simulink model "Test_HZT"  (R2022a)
settings: Solver=VariableStepAuto  StartTime=0.0  StopTime=10.0  RelTol=1e-3

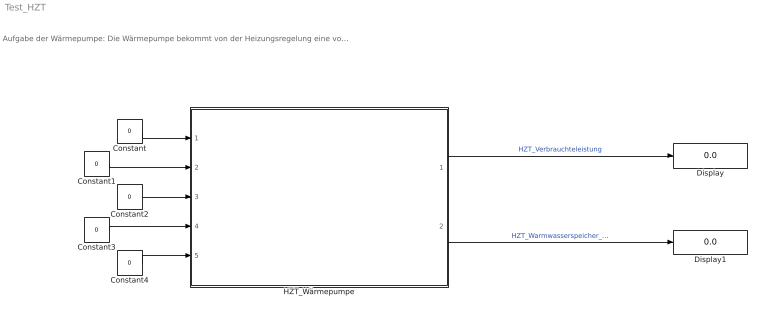
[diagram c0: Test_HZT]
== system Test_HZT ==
  note: Aufgabe der Wärmepumpe: Die Wärmepumpe bekommt von der Heizungsregelung eine vorgegebene Heizleistung, welche in das Haus eingespeist werden soll. Die Leistung wird dann von den Energieerzeugern genommen und umgewandelt. Das gleiche gilt für die Warmwasserheizleistung.
  Constant{,1..4} (5 alike) : Constant  Value=0
  Display : Display
  Display1 : Display
  HZT_Wärmepumpe : Subsystem
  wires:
  HZT_Wärmepumpe/1(HZT_verbrauchte_Leistung) -> Display/1  "HZT_Verbrauchteleistung"
  Constant1/1 -> HZT_Wärmepumpe/2(PAR_LKT_Temperatur)
  Constant4/1 -> HZT_Wärmepumpe/5(ESP_Stromnetz)
  HZT_Wärmepumpe/2(HZT_Warmwasserspeicher_verbrauchte_Leistung) -> Display1/1  "HZT_Warmwasserspeicher_verbrauchte_Leistung"
  Constant/1 -> HZT_Wärmepumpe/1(HZR_Heizleistung)
  Constant2/1 -> HZT_Wärmepumpe/3(HZR_Warmwasserleistung)
  Constant3/1 -> HZT_Wärmepumpe/4(ESP_Strom)

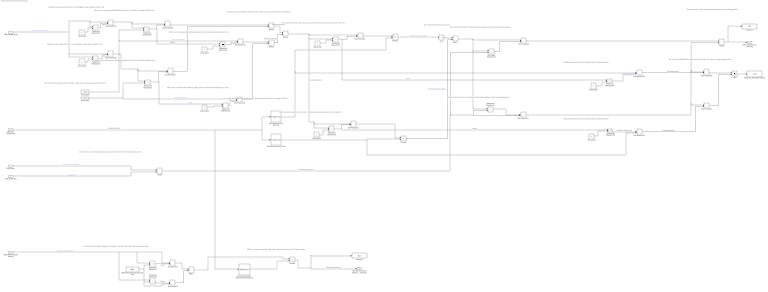
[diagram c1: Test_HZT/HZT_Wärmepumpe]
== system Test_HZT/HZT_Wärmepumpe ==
  note: Summiert alle Leistungen zusammen. (Es kommt nur aus einem Pfad ein tatsächlicher Wert, die anderen ergeben null)
  note: Modul zur berechnung der tatsächlich verbrauchten Energie für Warmwasser
  note: Leistung muss größer nulll sein, um anzugeben, dass geheizt werden soll
  note: Wenn gekühlt werden soll, wird die zu verbrauchende Leistung errechnet indem die Kühlleistung durch die Jahresarbeitszahl geteilt wird
  note: Die verbrauchte Leistung wird zusammengerechnet und angegeben
  note: Kontrolle der benötigen Energie im Vergleich mit der maximalen Wärmepumpen Energie für Warmwasser.
  note: Über die Temperatur ergibt sich die Jahresarbeitszahl, welche aussagt, wie Effizient die Wärmepumpe ist.
  note: Die maximal zu verbrauchende Leistung wird berechnet indem das gestzte Limit (variabel) für den Strom und das Stromnetz addiert werden.
  note: Von uns definierte Maximale Heiz-/kühl- Leistungen. (Können angepasst werden)
  note: Wenn die zu erbringende Kühlleistung kleiner ist als die maximale Kühlleistung, kann die angegebene Kühlleistung für die weitere Berechnung genutzt werden.
  note: Wenn die berechnete zu verbrauchende Leistung kleiner ist als die eingespeiste Leistung, kann die berechnete ausgegeben werden.
  note: Wenn die zu erbringende Leistung größer als die maximale Heizleistung ist, wird die maximale Heizleistung angenommen
  note: Die verbrauchte Kühlleistung wird
  note: Leistung muss kleiner nulll sein, um anzugeben, dass gekühlt werden soll
  note: Wenn die zu erbringende Heizleistung kleiner ist als die maximale Heizleistung, kann die angegebene Heizleistung für die weitere Berechnung genutzt werden.
  note: Wenn die berechnete zu verbrauchende Leistung größer ist als die eingespeiste Leistung, wird die maximale eingespeiste Leistung weiter genutzt.
  note: Die Jahresarbeitszahl für das Kühlen wird neu Übernommen
  note: Die Jahresarbeitszahl für das Heizen wird neu Übernommen
  note: Wenn geheizt werden soll, wird die zu verbrauchende Leistung errechnet indem die Heizleistung durch die Jahresarbeitszahl geteilt wird
  note: Wenn die zu erbringende Leistung kleiner als die maximale Kühlleistung ist, wird die maximale Kühlleistung angenommen
  note: Die neue Heiz-/Kühlleistung wird berechnet indem die maximal eingespeisste Energie mit den Jahresarbeitszahlen für entwedet Kühlen oder Heizen multipliziert wird. Und somit ergibt sich die maximale Heiz-/Kühlleistung, die die Wärmepumpe erbringen kann.
  HZR_Heizleistung : Inport
  PAR_LKT_Temperatur : Inport  Port=2
  HZR_Warmwasserleistung : Inport  Port=3
  ESP_Strom : Inport  Port=4
  ESP_Stromnetz : Inport  Port=5
  Abs1 : Abs
  Add{1,7..13} (8 alike) : Sum
  Display1 : Display
  Display2 : Display
  Divide1 : Product  Inputs=*/
  Divide2 : Product  Inputs=*/
  Divide3 : Product  Inputs=*/
  Dot Product{1..2,15..28} (16 alike) : DotProduct
  Jahresarbeitszahl_Heizen : Lookup_n-D  NumberOfTableDimensions=1  BreakpointsForDimension1=[-20;-15;-10;-5;0;5;10;20;30]  Table=[1.5;1.7;2.05;2.4;2.7;3;3.2;3.5;3.7]  InternalRulePriority=Speed  RndMeth=Simplest
  Jahresarbeitszahl_Kühlung : Lookup_n-D  NumberOfTableDimensions=1  BreakpointsForDimension1=[20;25;30;35;40]  Table=[3.7;3.2;2.8;2.2;1.5]  InternalRulePriority=Speed  RndMeth=Simplest
  Jahresarbeitszahl_Warmwassererhitzung : Lookup_n-D  NumberOfTableDimensions=1  BreakpointsForDimension1=[-20;-15;-10;-5;0;5;10;15;20;25;30;35;40]  Table=[2.2;2.4;2.6;2.8;2.9;3;3.2;3.5;4;4.5;5;5.5;6]  InternalRulePriority=Speed  RndMeth=Simplest
  Leistung{12..17,21..22} (8 alike) : Constant  Value=0
  Leistung18 : Constant  Value=10000
  Leistung19 : Constant  Value=-10000
  Maximale Heiz/Kühlleistung : Display
  Maximale Warmwasser-Leistung : Constant  Value=4500
  Relational Operator{1,13..14,16,21} (5 alike) : RelationalOperator  Operator=<  OutDataTypeStr=boolean  RndMeth=Simplest
  Relational Operator{2,12,15,17,20} (5 alike) : RelationalOperator  Operator=>  OutDataTypeStr=boolean  RndMeth=Simplest
  Relational Operator18 : RelationalOperator  Operator=~=  OutDataTypeStr=boolean  RndMeth=Simplest
  Relational Operator19 : RelationalOperator  Operator=~=  OutDataTypeStr=boolean  RndMeth=Simplest
  Relational Operator22 : RelationalOperator  Operator===  OutDataTypeStr=boolean  RndMeth=Simplest
  Relational Operator23 : RelationalOperator  Operator===  OutDataTypeStr=boolean  RndMeth=Simplest
  HZT_verbrauchte_Leistung : Outport
  HZT_Warmwasserspeicher_verbrauchte_Leistung : Outport  Port=2
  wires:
  Add10/1 -> Add12/1  "Benötigte Leistung"
  Relational Operator2/1 -> Dot Product2/1  "Heizen"
  Relational Operator23/1 -> Dot Product18/2  "Heizen"
  Relational Operator19/1 -> Dot Product25/1  "Benötigte Kühlleistung"
  Dot Product23/1 -> Add13/2, Dot Product26/1, Dot Product27/1
  Leistung14/1 -> Relational Operator15/2
  Dot Product16/1 -> Add10/2
  Dot Product26/1 -> Add9/1
  Dot Product25/1 -> Dot Product27/2  "jahresarbeitszahl"
  Relational Operator12/1 -> Dot Product15/2, Relational Operator19/1  "Heizen"
  Leistung12/1 -> Relational Operator12/2
  Relational Operator16/1 -> Dot Product22/2
  Dot Product1/1 -> Add1/1
  Abs1/1 -> Add7/1
  Relational Operator13/1 -> Relational Operator18/1, Dot Product21/2  "Kühlen"
  Add11/1 -> Add12/2  "Benötigte Leistung"
  Relational Operator22/1 -> Dot Product17/2  "Kühlen"
  Add9/1 -> Maximale Heiz/Kühlleistung/1
  Dot Product18/1 -> Add11/2
  Dot Product19/1 -> Relational Operator20/1, Dot Product28/1
  Dot Product22/1 -> Add13/1
  HZR_Warmwasserleistung/1 -> Relational Operator1/1, Dot Product1/1, Relational Operator2/1  "Benötigte Leistung Warmwsser"
  Dot Product27/1 -> Add9/2
  Leistung22/1 -> Relational Operator23/2
  Relational Operator14/1 -> Dot Product19/2  "Kühlen"
  Relational Operator18/1 -> Dot Product24/2  "Benötigte Kühlleistung"
  Relational Operator15/1 -> Dot Product20/2  "Heizen"
  Jahresarbeitszahl_Heizen/1 -> Dot Product25/2, Divide2/2
  Relational Operator17/1 -> Dot Product23/1
  Add1/1 -> Divide1/1
  Relational Operator20/1 -> Relational Operator22/1, Dot Product28/2  "Kühlen"
  Leistung17/1 -> Relational Operator19/2
  Leistung13/1 -> Relational Operator14/2
  HZR_Heizleistung/1 -> Dot Product19/1, Relational Operator14/1, Relational Operator15/1, Dot Product20/1  "Benötigte Leistung Heizen"
  Leistung18/1 -> Dot Product18/1, Relational Operator21/2  "maximale Leistung"
  ESP_Stromnetz/1 -> Add8/2  "Leistung Netz"
  Dot Product24/1 -> Dot Product26/2  "jahresarbeitszahl"
  Dot Product20/1 -> Relational Operator21/1, Dot Product16/1
  Add8/1 -> Relational Operator16/2, Dot Product23/2, Relational Operator17/2  "Eingespeiste Leistung"
  Dot Product28/1 -> Add10/1
  Dot Product17/1 -> Add11/1
  Add13/1 -> Display2/1, HZT_verbrauchte_Leistung/1
  Leistung21/1 -> Relational Operator22/2
  Leistung19/1 -> Relational Operator20/2, Dot Product17/1  "maximale Leistung"
  Jahresarbeitszahl_Kühlung/1 -> Divide3/2, Dot Product24/1
  Dot Product15/1 -> Divide2/1
  Relational Operator1/1 -> Dot Product1/2  "Heizen"
  Jahresarbeitszahl_Warmwassererhitzung/1 -> Divide1/2
  ESP_Strom/1 -> Add8/1  "Leistung Strom (Speicher/PV)"
  Leistung16/1 -> Relational Operator18/2
  Maximale Warmwasser-Leistung/1 -> Relational Operator1/2, Dot Product2/2, Relational Operator2/2
  Add7/1 -> Dot Product22/1, Relational Operator16/1, Relational Operator17/1
  Divide3/1 -> Abs1/1  "Zu_Verbrauchende_Kühlleistung"
  Dot Product2/1 -> Add1/2
  Dot Product21/1 -> Divide3/1
  Leistung15/1 -> Relational Operator13/2
  PAR_LKT_Temperatur/1 -> Jahresarbeitszahl_Warmwassererhitzung/1, Jahresarbeitszahl_Heizen/1, Jahresarbeitszahl_Kühlung/1  "Außentemperatur"
  Divide1/1 -> Display1/1, HZT_Warmwasserspeicher_verbrauchte_Leistung/1  "Warmwasserleistung"
  Add12/1 -> Dot Product21/1, Dot Product15/1, Relational Operator12/1, Relational Operator13/1  "Benötigte Leistung"
  Divide2/1 -> Add7/2  "Zu_Verbrauchende_Heizleistung"
  Relational Operator21/1 -> Dot Product16/2, Relational Operator23/1  "Heizen"
